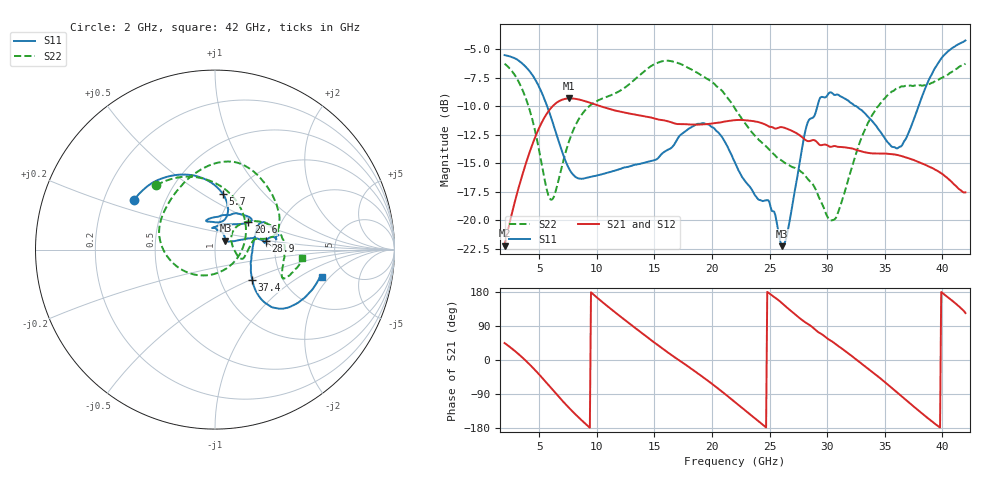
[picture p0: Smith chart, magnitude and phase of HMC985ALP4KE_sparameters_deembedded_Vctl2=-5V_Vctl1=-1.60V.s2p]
!s2p File: Measurements: S11, S21, S12, S22
# GHz S dB R 50.0
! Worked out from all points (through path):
!   401 points, 2 GHz to 42 GHz, reference 50 ohm
!   highest |S21| = -9.33 dB at 7.6 GHz (marker M1); lowest = -22.3 dB at 2 GHz (marker M2)
!   lowest |S11| = -22.3 dB at 26.1 GHz (marker M3), VSWR 1.17, Z = 55.9 + j5.63 ohm
!   |S11| at or under -10 dB: 5.687 GHz to 29.15 GHz (23.47 GHz wide, 135 % of centre); 32.5 GHz to 37.94 GHz (5.436 GHz wide, 15.4 % of centre)
!   |S22| runs from -20.0 to -6.0 dB; largest |S21 - S12| = 0.00034
!   S11 on the Smith chart (normalised r, x): 2 GHz: 0.33, +0.25; 5.7 GHz: 0.89, +0.62; 20.6 GHz: 1.37, +0.45; 28.9 GHz: 1.78, +0.19; 37.4 GHz: 1.42, -0.51; 42 GHz: 3.30, -1.64
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2  -5.53 148.6  -22.26 44.7  -22.27 44.7  -6.28 132.4
3.6  -6.33 122.2  -15.84 5.0  -15.84 5.0  -8.70 88.8
4.7  -7.75 101.2  -12.61 -28.3  -12.61 -28.3  -12.42 46.7
5.7  -10.04 82.2  -10.61 -62.3  -10.62 -62.3  -17.48 -19.8
6.3  -11.83 74.0  -9.89 -83.2  -9.89 -83.2  -17.90 -77.1
7.6  -15.51 73.8  -9.33 -126.5  -9.33 -126.5  -13.06 -151.6
8.7  -16.38 87.2  -9.49 -159.5  -9.49 -159.5  -10.74 179.1
12.1  -15.49 107.0  -10.51 113.6  -10.51 113.6  -8.61 132.0
15.4  -14.48 81.9  -11.19 37.1  -11.20 37.2  -6.15 84.0
17.9  -12.05 50.8  -11.60 -16.5  -11.61 -16.4  -6.63 55.2
20.6  -12.37 39.5  -11.46 -76.9  -11.47 -76.9  -8.41 20.2
22  -14.95 52.2  -11.23 -111.3  -11.24 -111.3  -10.21 12.1
24  -18.17 92.4  -11.40 -160.6  -11.40 -160.6  -12.89 14.5
26.1  -22.29 40.7  -11.86 149.3  -11.86 149.3  -14.81 -2.9
28.7  -11.05 7.6  -12.99 87.1  -13.00 87.1  -16.77 -18.1
28.9  -10.85 9.8  -13.00 81.7  -13.00 81.8  -17.12 -17.3
30.7  -9.03 15.0  -13.51 42.7  -13.51 42.7  -19.89 25.5
33.2  -10.56 30.5  -14.04 -14.4  -14.05 -14.3  -12.26 40.1
35.4  -13.32 8.0  -14.19 -68.3  -14.19 -68.2  -8.93 18.3
37.4  -11.50 -38.8  -14.70 -119.9  -14.70 -119.9  -8.24 -3.4
39.7  -6.12 -41.8  -15.76 -176.1  -15.76 -176.1  -7.67 -23.1
42  -4.25 -14.6  -17.57 123.9  -17.57 123.9  -6.27 -5.6
